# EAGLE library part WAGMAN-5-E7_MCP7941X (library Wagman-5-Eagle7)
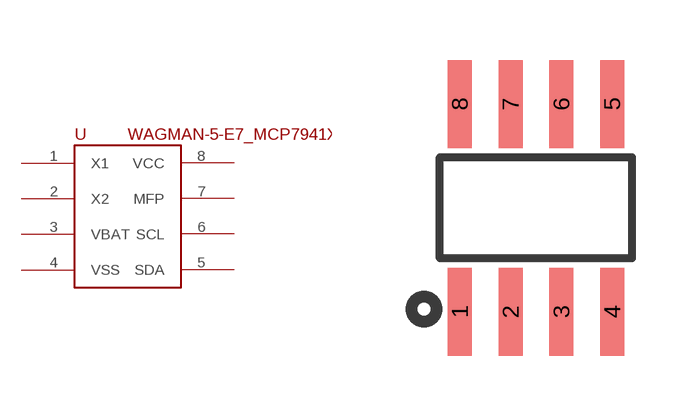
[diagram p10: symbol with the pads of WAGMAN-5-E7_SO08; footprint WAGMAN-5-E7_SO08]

Designator prefix U

## WAGMAN-5-E7_MCP7941X-SOIC-8  [WAGMAN-5-E7_SO08]
1  X1  pas
2  X2  pas
3  VBAT  pas
4  VSS  pas
5  SDA  pas
6  SCL  pas
7  MFP  pas
8  VCC  pas

## Footprint WAGMAN-5-E7_SO08 (pad centres in mm)
SMALL OUTLINE INTEGRATED CIRCUIT body 3.9 mm/JEDEC MS-012AA
smd 0.6 x 2.2: 1 -1.905,-2.6; 2 -0.635,-2.6; 3 0.635,-2.6; 4 1.905,-2.6; 5 1.905,2.6; 6 0.635,2.6; 7 -0.635,2.6; 8 -1.905,2.6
